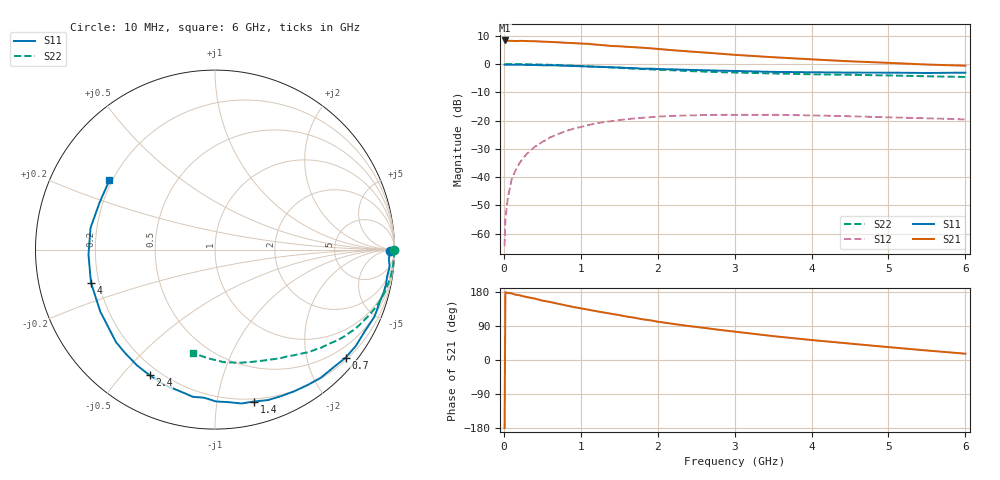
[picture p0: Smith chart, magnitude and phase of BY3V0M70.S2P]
! SIEMENS Small Signal Semiconductors
! BFY420
! Si NPN RF SIEGET Grounded Emitter Transistor in MICRO-X
! VCE = 3 V  IC = 0.7 mA
! Common Emitter S-Parameters:  October  1996
# GHz  S  MA  R  50
!  f  S11  S21  S12  S22
! GHz  MAG  ANG  MAG  ANG  MAG  ANG  MAG  ANG
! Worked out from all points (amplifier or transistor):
!   36 points, 10 MHz to 6 GHz, reference 50 ohm
!   highest |S21| = 8.3 dB at 10 MHz (marker M1)
!   |S21| within 3 dB of that: start of sweep to 2.002 GHz
!   unconditionally stable (mu >= 1): 4.656 GHz to end of sweep
!   at 250 MHz: K = 0.04, MSG = 20.7 dB, |S12| = -33.3 dB
!   at 1.4 GHz: K = 0.17, MSG = 13.3 dB, |S12| = -20.2 dB
!   at 6 GHz: K = 1.38, MAG = 5.8 dB, |S12| = -19.6 dB
!   S11 on the Smith chart (normalised r, x): 10 MHz: 65, -25; 700 MHz: 0.25, -2.76; 1.4 GHz: 0.18, -1.27; 2.4 GHz: 0.16, -0.60; 4 GHz: 0.17, -0.13; 6 GHz: 0.19, +0.29
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0.01  0.9735 -0.6  2.612 -179.3  0.0006 121.0  0.9999 -0.2
0.02  0.9746 -1.4  2.606 178.8  0.0018 91.9  0.9991 -0.6
0.05  0.97 -2.9  2.564 177.2  0.0041 88.1  0.9993 -1.4
0.1  0.9775 -5.7  2.574 175.9  0.009 87.1  0.9962 -2.7
0.15  0.9708 -8.6  2.548 172.4  0.013 83.7  0.9963 -4.1
0.25  0.9697 -14.4  2.564 168.4  0.0216 80.2  0.9933 -6.6
0.4  0.9637 -22.9  2.53 162.3  0.0341 76.3  0.9851 -10.6
0.5  0.9504 -28.7  2.492 156.7  0.0418 72.9  0.9775 -13.2
0.7  0.9444 -39.6  2.426 148.7  0.0574 65.9  0.958 -18.2
0.9  0.9258 -50.4  2.344 140.0  0.0715 59.1  0.9343 -22.9
1.1  0.9038 -61.1  2.272 132.7  0.0835 52.9  0.908 -27.5
1.4  0.8738 -75.6  2.085 121.9  0.0976 44.2  0.8697 -33.6
1.6  0.8528 -85.1  2.019 114.5  0.1059 38.8  0.8408 -37.5
1.8  0.8276 -94.1  1.943 107.5  0.1118 34.2  0.8163 -40.8
2.2  0.8045 -110.4  1.754 95.4  0.1212 25.2  0.7751 -47.4
2.4  0.7891 -117.5  1.673 89.7  0.1232 21.8  0.7514 -50.5
2.8  0.7638 -130.8  1.529 79.6  0.1264 15.0  0.7181 -56.0
3.5  0.7264 -151.6  1.32 63.0  0.1265 6.0  0.6806 -64.8
4  0.7152 -165.1  1.21 52.7  0.1235 1.2  0.6597 -71.3
4.5  0.7054 -177.8  1.117 43.3  0.1191 -2.6  0.6452 -77.9
5.5  0.6945 158.1  0.979 25.1  0.1097 -5.8  0.6075 -93.2
6  0.7041 146.6  0.934 16.6  0.1048 -5.0  0.5903 -101.8
